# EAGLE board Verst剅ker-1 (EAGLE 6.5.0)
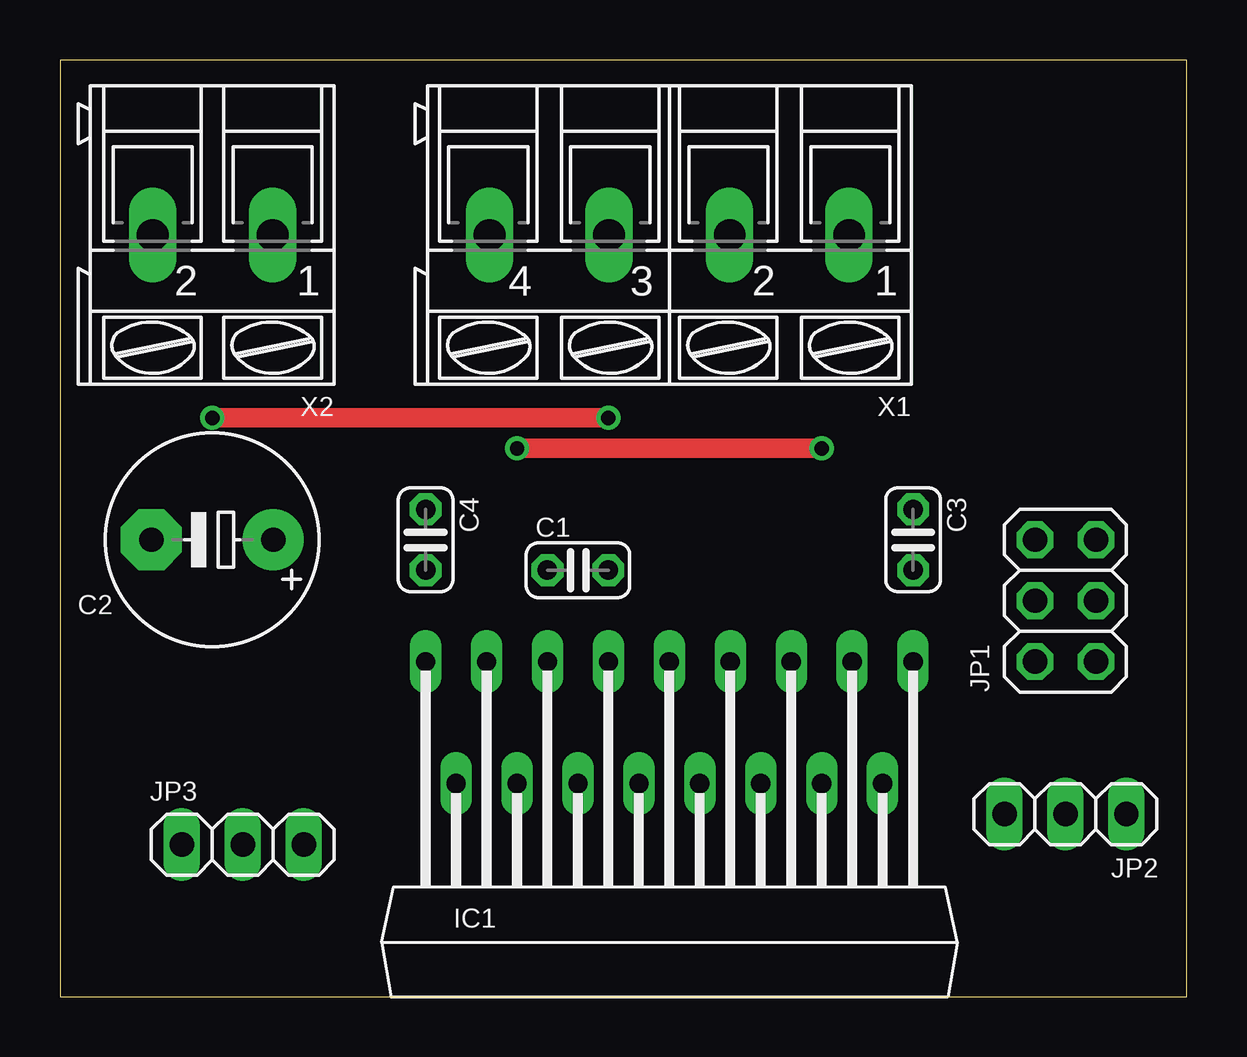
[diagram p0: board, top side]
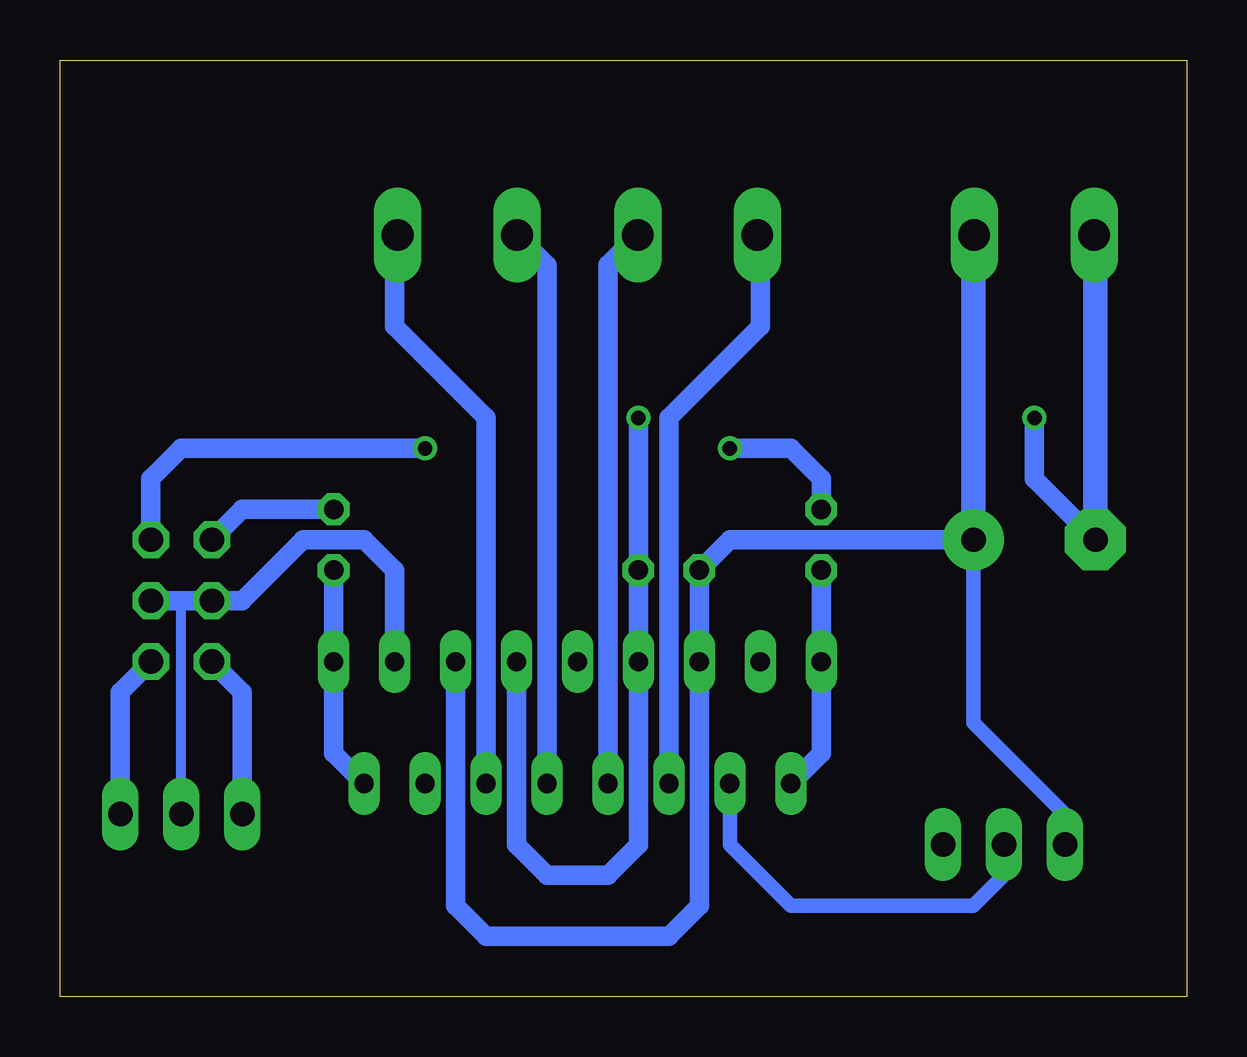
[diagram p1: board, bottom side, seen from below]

Size 46.97 x 39.04 mm. Coordinates in mm from the lower left corner, seen from the top.
Outline: 0,0 46.97,0 46.97,39.04 0,39.04 0,0
Copper layers (1*16): Top 0.035mm / dielectric 1.5mm / Bottom 0.035mm
Design rules "default": minimum track width 10mil, minimum drill 24mil, track to track 8mil, track to pad 8mil, pad to pad 8mil, via to via 8mil, smd to smd 8mil, copper to edge 40mil, drill to drill 8mil, minimum pad ring 10mil, minimum via ring 8mil, stop-mask expansion 4mil, vias tented up to drill 0mil, thermal gap 10mil

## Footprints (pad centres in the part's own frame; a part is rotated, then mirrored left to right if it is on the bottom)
C025-024X044 = drill 0.813 octagon: 1 -1.27,0; 2 1.27,0
E5-8,5 = drill 1.016 pad 2.54: + -2.54,0 | drill 1.016 pad 2.54 octagon: - 2.54,0
SOT243-1 = drill 0.8 long: 1 10.16,13.97; 2 8.89,8.89; 3 7.62,13.97; 4 6.35,8.89; 5 5.08,13.97; 6 3.81,8.89; 7 2.54,13.97; 8 1.27,8.89; 9 0,13.97; 10 -1.27,8.89; 11 -2.54,13.97; 12 -3.81,8.89; 13 -5.08,13.97; 14 -6.35,8.89; 15 -7.62,13.97; 16 -8.89,8.89; 17 -10.16,13.97
2X03 = drill 1.016 octagon: 1 -2.54,-1.27; 2 -2.54,1.27; 3 0,-1.27; 4 0,1.27; 5 2.54,-1.27; 6 2.54,1.27
1X03 = drill 1.016 long: 1 -2.54,0; 2 0,0; 3 2.54,0
AK300/4 = drill 1.321 long: 1 -7.493,0; 2 -2.515,0; 3 2.515,0; 4 7.493,0
AK300/2 = drill 1.321 long: 1 -2.515,0; 2 2.489,0

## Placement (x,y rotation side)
C1  100n  [C025-024X044]  21.59,17.78 0 top
C2  2200µF  [E5-8,5]  6.35,19.05 180 top
C3  220n  [C025-024X044]  35.56,19.05 270 top
C4  220n  [C025-024X044]  15.24,19.05 270 top
IC1  TDA1558  [SOT243-1]  25.4,0 0 top
JP1  Lautstärke  [2X03]  41.91,16.51 90 top
JP2  Signaleingang  [1X03]  41.91,7.62 180 top
JP3  Stummschalter  [1X03]  7.62,6.35 0 top
X1  Lautsprecher  [AK300/4]  25.4,31.75 180 top
X2  Spannungsversorgung  [AK300/2]  6.35,31.75 180 top

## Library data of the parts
C1-C4 = rcl
IC1 = Audio-Power-amplifier
JP1-JP3 = pinhead
X1 X2 = con-ptr500; OC_FARNELL: unknown; OC_NEWARK: unknown

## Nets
+12V: C1.1 C2.+ IC1.5 IC1.13 JP3.1 X2.1
GND: C1.2 C2.- IC1.7 IC1.11 X2.2
N$1: C3.2 IC1.1 IC1.2
N$2: C4.2 IC1.16 IC1.17
N$3: JP1.2 JP2.3
N$4: JP1.1 JP2.1
N$5: IC1.6 X1.1
N$6: IC1.8 X1.2
N$7: IC1.3 JP1.3 JP1.4 JP2.2
N$8: IC1.10 X1.3
N$9: IC1.12 X1.4
N$10: C4.1 JP1.5
N$11: C3.1 JP1.6
N$12: IC1.14 JP3.2

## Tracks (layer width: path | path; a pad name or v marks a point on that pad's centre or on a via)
+12V
  Bottom 0.61: C2.+ 8.89,11.43 5.08,7.62 JP3.1
  Bottom 0.813: C2.+ 19.05,19.05 C1.1 IC1.13 20.32,3.81 21.59,2.54 29.21,2.54 30.48,3.81 IC1.5
  Bottom 1.016: X2.1 8.89,31.75 C2.+
GND  (via drill 0.6)
  Top 0.813: v6.35,24.13 v22.86,24.13
  Bottom 0.813: IC1.7 27.94,6.35 26.67,5.08 24.13,5.08 22.86,6.35 IC1.11 C1.2 v22.86,24.13 | C2.- 6.35,21.59 v6.35,24.13
  Bottom 1.016: X2.2 3.81,31.75 C2.-
N$1
  Bottom 0.813: IC1.2 35.56,10.16 IC1.1 C3.2
N$2
  Bottom 0.813: C4.2 IC1.17 15.24,10.16 IC1.16
N$3
  Bottom 0.813: JP2.3 39.37,12.7 JP1.2
N$4
  Bottom 0.813: JP2.1 44.45,12.7 JP1.1
N$5
  Bottom 0.813: IC1.6 29.21,24.13 33.02,27.94 33.02,31.62 X1.1
N$6
  Bottom 0.813: IC1.8 26.67,30.48 27.94,31.75 27.94,31.73 X1.2
N$7
  Bottom 0.406: JP2.2 41.91,16.51
  Bottom 0.813: IC1.3 33.02,17.78 34.29,19.05 36.83,19.05 39.37,16.51 JP1.4 41.91,16.51 JP1.3
N$8
  Bottom 0.813: IC1.10 24.13,30.5 X1.3
N$9
  Bottom 0.813: IC1.12 21.59,24.13 17.78,27.94 17.78,31.62 X1.4
N$10  (via drill 0.6)
  Top 0.813: v19.05,22.86 v31.75,22.86
  Bottom 0.813: C4.1 15.24,21.59 16.51,22.86 v19.05,22.86 | v31.75,22.86 41.91,22.86 43.18,21.59 JP1.5
N$11
  Bottom 0.813: JP1.6 39.37,20.32 C3.1
N$12
  Bottom 0.61: IC1.14 19.05,6.35 16.51,3.81 8.89,3.81 7.62,5.08 JP3.2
